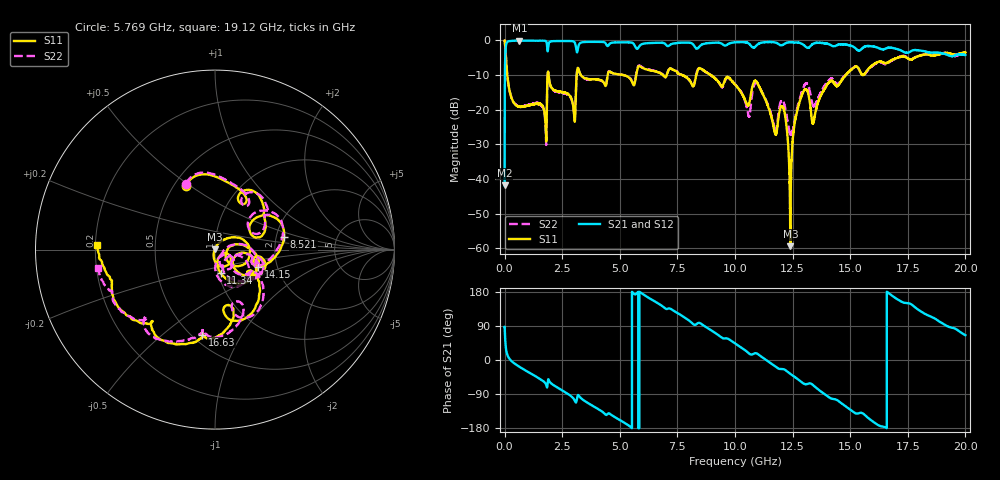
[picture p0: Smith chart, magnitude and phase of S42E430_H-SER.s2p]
!{S42E430}
!Johanson Technology Inc.
!www.johansontechnology.com
!Test Board Conditions:
!Substrate Type  RO4350B
!Substrate Thickness  50 mil
!Substrate Dk  3.66
!TL Type: GCPW
!TL Trace Width  60 mil
!TL Gap  10 mil
!Electrode orientation  Horizontal
!DUT TOPOLOGY	SERIES
!Mounting Pad LxW  14x55 mil
! Created Wed Nov 25 22:16:11 2020
# khz S ma R 50
! 2 Port Network Data from SP1.SP block
! freq  magS11  angS11  magS21  angS21  magS12  angS12  magS22  angS22
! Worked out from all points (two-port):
!   20001 points, 300 kHz to 20 GHz, reference 50 ohm
!   highest |S21| = -0.07 dB at 643.3 MHz (marker M1); lowest = -41.9 dB at 300 kHz (marker M2)
!   |S21| within 3 dB of the highest: 37.06 MHz to 1.862 GHz (1.825 GHz wide, 192 % of centre); 3.165 GHz to 17.25 GHz (14.09 GHz wide, 138 % of centre)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
!   lowest |S11| = -59.4 dB at 12.4 GHz (marker M3), VSWR 1.00, Z = 49.9 + j0.0718 ohm
!   |S11| at or under -10 dB: 114.8 MHz to 1.867 GHz (1.752 GHz wide, 177 % of centre); 1.911 GHz to 3.13 GHz (1.219 GHz wide, 48.4 % of centre); 8.944 GHz to 14.81 GHz (5.869 GHz wide, 49.4 % of centre)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
!   |S22| runs from -30.2 to 0.0 dB; largest |S21 - S12| = 0.019
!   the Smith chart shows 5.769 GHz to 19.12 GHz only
!   S11 on the Smith chart (normalised r, x): 5.769 GHz: 0.58, +0.48; 8.521 GHz: 2.21, +0.37; 11.34 GHz: 1.03, -0.27; 14.15 GHz: 1.59, -0.33; 16.63 GHz: 0.56, -0.69; 19.12 GHz: 0.21, +0.02
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300  0.9967 -0.6  0.008041 87.9  0.008072 89.2  0.9944 -0.7
118300  0.3086 -76.6  0.9499 13.6  0.9507 13.5  0.3094 -76.5
643300  0.1101 -109.5  0.9924 -17.9  0.9911 -17.9  0.1113 -108.3
1733300  0.09101 -144.2  0.9898 -58.7  0.9897 -58.7  0.08692 -145.9
1945300  0.2566 -142.6  0.9469 -56.4  0.9466 -56.5  0.2528 -142.2
2988300  0.1059 174.2  0.9693 -101.6  0.9685 -101.5  0.1045 -175.2
3334300  0.3077 167.3  0.9343 -101.7  0.9347 -101.7  0.3047 173.6
5769300  0.3881 114.6  0.7572 178.2  0.7573 178.2  0.4011 113.5
6667300  0.3466 61.7  0.9262 149.2  0.9228 149.1  0.3505 59.8
8521300  0.3914 10.5  0.8559 95.9  0.8529 95.8  0.3917 14.5
1.00003e7  0.2316 -39.4  0.9381 44.0  0.9383 44.1  0.2322 -49.1
1.13383e7  0.135 -75.9  0.9456 0.4  0.9463 0.5  0.1383 -86.8
1.17423e7  0.04581 -56.5  0.9345 -16.8  0.9354 -16.8  0.0488 -61.2
1.21003e7  0.1055 -63.9  0.8712 -24.2  0.8741 -24.3  0.1304 -57.6
1.24013e7  0.001067 137.7  0.9415 -36.5  0.9431 -36.7  0.04451 -39.7
1.29033e7  0.1637 20.8  0.8976 -59.0  0.8949 -59.2  0.1822 6.4
1.33343e7  0.07277 -34.3  0.8665 -63.7  0.8649 -63.7  0.1316 -45.8
1.41533e7  0.2594 -22.2  0.8551 -101.0  0.857 -100.6  0.2805 -26.4
1.66343e7  0.4791 -98.5  0.7815 178.4  0.7723 178.3  0.4672 -98.7
1.66673e7  0.4863 -98.4  0.7887 176.9  0.7736 176.6  0.4769 -99.8
1.91203e7  0.6595 177.5  0.6351 92.6  0.6387 92.3  0.661 -171.3
2e7  0.6724 154.2  0.6128 65.3  0.6124 66.3  0.6617 160.3
